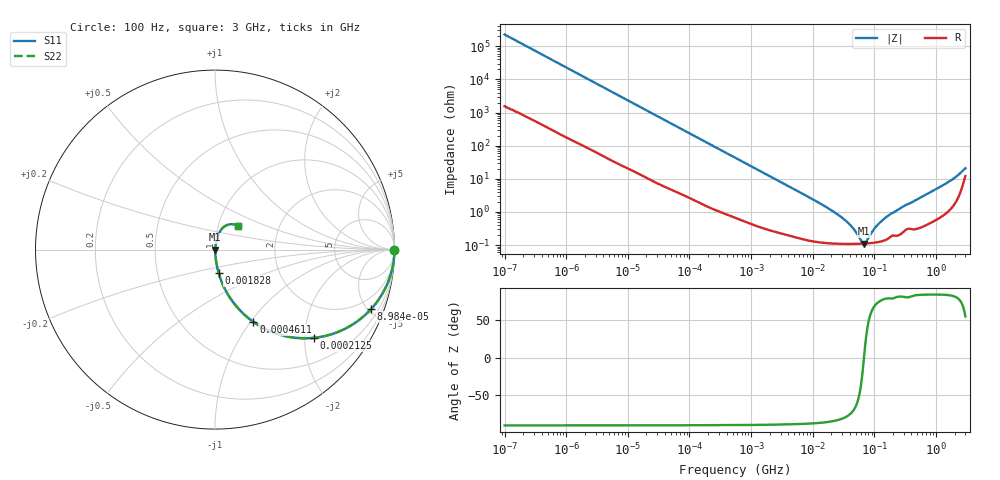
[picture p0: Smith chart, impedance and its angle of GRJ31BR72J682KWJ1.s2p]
!Murata Part Number: GRJ31BR72J682KWJ1
!These Parameters are Measured in Series Mode Connection
!Data Generated on Jun 19, 2026
!  o--ll--o
!Port1  Port2
!  o------o
!Operation Temp=25[degC], DC Bias Voltage=0[V]
!Freq. Start=100[Hz] Stop=3[GHz] 401[Steps]
# Hz S RI R 50
!Freq.(Hz) S11(Real) S11(Imag) S21(Real) S21(Imag) S12(Real) S12(Imag) S22(Real) S22(Imag)
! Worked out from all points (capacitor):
!   401 points, 100 Hz to 3 GHz, reference 50 ohm
!   read as one part in series: C = 7.01 nF near 109 Hz
!   lowest |Z| = 111 mohm at 67.94 MHz (marker M1)
!   series resonance near 67.85 MHz, so ESL is about 790 pH
!   S11 on the Smith chart (normalised r, x): 100 Hz: open; 89.84 kHz: 1.06, -5.24; 212.5 kHz: 1.03, -2.23; 461.1 kHz: 1.02, -1.03; 1.828 MHz: 1.01, -0.26; 3 GHz: 1.24, +0.34
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100  1 -0.000441  3.2e-06 0.000441  3.2e-06 0.000441  1 -0.000441
1788  0.9999 -0.00777  0.000123 0.00777  0.000123 0.00777  0.9999 -0.00777
10443  0.9976 -0.0448  0.00241 0.0448  0.00241 0.0448  0.9976 -0.0448
31977  0.9804 -0.1339  0.0196 0.1339  0.0196 0.1339  0.9804 -0.1339
89839  0.8701 -0.3307  0.1299 0.3307  0.1299 0.3307  0.8701 -0.3307
138163  0.7425 -0.4315  0.2575 0.4315  0.2575 0.4315  0.7425 -0.4315
212480  0.5533 -0.4911  0.4467 0.4911  0.4467 0.4911  0.5533 -0.4911
461094  0.2139 -0.4028  0.7861 0.4028  0.7861 0.4028  0.2139 -0.4028
547723  0.1631 -0.3618  0.8369 0.3618  0.8369 0.3618  0.1631 -0.3618
918067  0.0675 -0.2422  0.9325 0.2422  0.9325 0.2422  0.0675 -0.2422
1827928  0.0198 -0.1288  0.9802 0.1288  0.9802 0.1288  0.0198 -0.1288
9794414  0.0019 -0.0245  0.9981 0.0245  0.9981 0.0245  0.0019 -0.0245
2.035898e7  0.00124 -0.011  0.9988 0.011  0.9988 0.011  0.00124 -0.011
3.268714e7  0.00112 -0.00578  0.9989 0.00578  0.9989 0.00578  0.00112 -0.00578
4.418008e7  0.00109 -0.00321  0.9989 0.00321  0.9989 0.00321  0.00109 -0.00321
6.234031e7  0.0011 -0.000615  0.9989 0.000615  0.9989 0.000615  0.0011 -0.000615
6.794454e7  0.00111 1.08e-05  0.9989 -1.08e-05  0.9989 -1.08e-05  0.00111 1.08e-05
7.405258e7  0.00112 0.000637  0.9989 -0.000637  0.9989 -0.000637  0.00112 0.000637
1.090876e8  0.00122 0.00359  0.9988 -0.00359  0.9988 -0.00359  0.00122 0.00359
1.751444e8  0.00173 0.00801  0.9983 -0.00801  0.9983 -0.00801  0.00173 0.00801
1.71441e9  0.019 0.0842  0.981 -0.0842  0.981 -0.0842  0.019 0.0842
3e9  0.1282 0.1319  0.8718 -0.1319  0.8718 -0.1319  0.1282 0.1319
